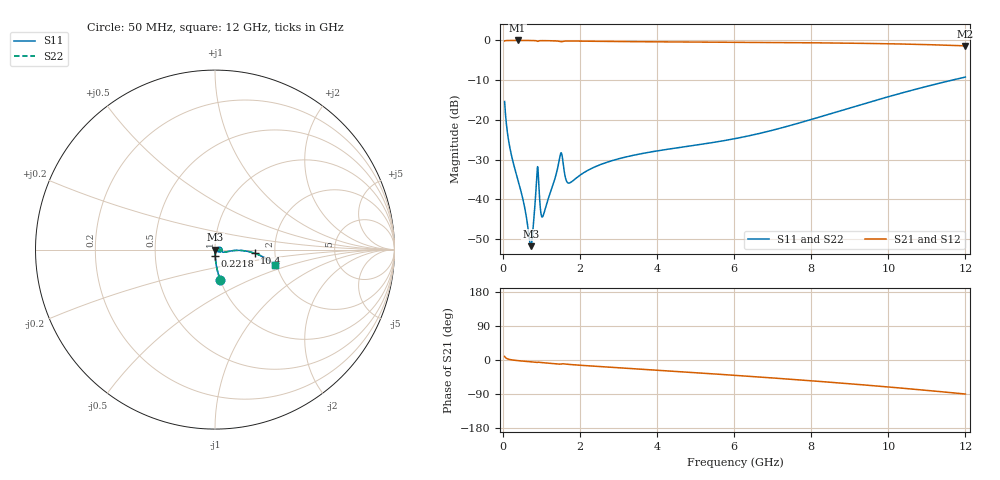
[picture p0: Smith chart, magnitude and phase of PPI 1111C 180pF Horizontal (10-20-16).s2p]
# MHz S MA R 50
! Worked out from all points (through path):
!   1601 points, 50 MHz to 12 GHz, reference 50 ohm
!   highest |S21| = -0.01 dB at 386.1 MHz (marker M1); lowest = -1.4 dB at 12 GHz (marker M2)
!   group delay of S21, straight-line fit = 20.3 ps
!   lowest |S11| = -51.8 dB at 729.7 MHz (marker M3), VSWR 1.01, Z = 50.2 - j0.0877 ohm
!   |S11| at or under -10 dB: start of sweep to 11.65 GHz
!   |S22| runs from -51.8 to -9.2 dB; largest |S21 - S12| = 0
!   S11 on the Smith chart (normalised r, x): 50 MHz: 1.00, -0.35; 221.8 MHz: 1.00, -0.07; 10.4 GHz: 1.56, -0.07; 12 GHz: 1.95, -0.39
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50  0.1702 -80.4  0.9849 9.5  0.9849 9.5  0.1702 -80.4
221.7812  0.03682 -88.5  0.9987 0.6  0.9987 0.6  0.03682 -88.5
386.0938  0.01814 -89.6  0.9992 -1.6  0.9992 -1.6  0.01814 -89.6
557.875  0.00845 -85.7  0.9988 -3.3  0.9988 -3.3  0.00845 -85.7
692.3125  0.003152 -53.8  0.9979 -4.5  0.9979 -4.5  0.003152 -53.8
729.6562  0.002569 -19.8  0.9975 -4.9  0.9975 -4.9  0.002569 -19.8
781.9375  0.003978 26.7  0.9966 -5.4  0.9966 -5.4  0.003978 26.7
856.625  0.01161 42.3  0.9922 -6.3  0.9922 -6.3  0.01161 42.3
893.9688  0.02334 18.0  0.9787 -6.6  0.9787 -6.6  0.02334 18.0
931.3125  0.01749 -39.4  0.9853 -5.7  0.9853 -5.7  0.01749 -39.4
998.5312  0.006387 -23.8  0.9938 -6.6  0.9938 -6.6  0.006387 -23.8
1043.344  0.006127 1.7  0.9939 -7.1  0.9939 -7.1  0.006127 1.7
1498.938  0.0372 10.0  0.9651 -10.9  0.9651 -10.9  0.0372 10.0
1693.125  0.01607 -13.4  0.9838 -11.4  0.9838 -11.4  0.01607 -13.4
2044.156  0.02071 3.0  0.9801 -14.1  0.9801 -14.1  0.02071 3.0
2813.438  0.03041 -5.5  0.9703 -19.2  0.9703 -19.2  0.03041 -5.5
4038.312  0.0409 -16.4  0.9596 -27.2  0.9596 -27.2  0.0409 -16.4
6025  0.05803 -13.8  0.9475 -40.5  0.9475 -40.5  0.05803 -13.8
8019.156  0.1017 -3.1  0.9336 -55.0  0.9336 -55.0  0.1017 -3.1
10013.31  0.1963 -3.8  0.9079 -71.3  0.9079 -71.3  0.1963 -3.8
10401.69  0.2214 -5.3  0.9001 -74.7  0.9001 -74.7  0.2214 -5.3
12000  0.3457 -14.6  0.8535 -89.8  0.8535 -89.8  0.3457 -14.6
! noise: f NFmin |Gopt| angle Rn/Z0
50  0.0004721  0.8929  0.4018  0.0009606
1372  0.0134  0.8968  9.248  0.02818
2701  0.02675  0.8998  18.09  0.05697
4031  0.03864  0.8993  26.69  0.07941
5360  0.04821  0.8966  34.98  0.09261
6682  0.05666  0.895  42.84  0.1021
8012  0.06474  0.8952  50.33  0.1105
9341  0.07281  0.897  57.38  0.119
1.067e+04  0.0812  0.9004  63.97  0.1284
1.2e+04  0.09017  0.9048  70.12  0.1394
